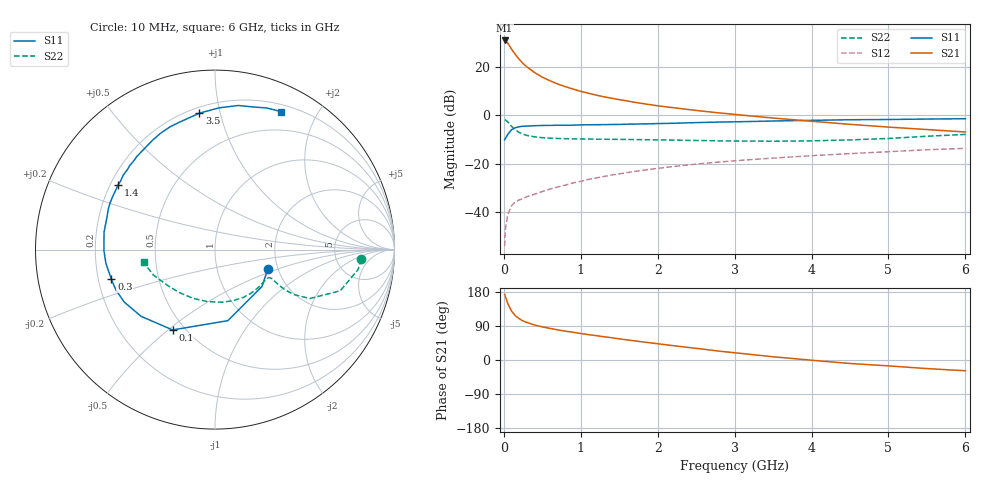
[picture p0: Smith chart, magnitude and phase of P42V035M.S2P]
! SIEMENS Small Signal Semiconductors
! BFP182
! Si NPN RF Bipolar Junction Transistor in SOT143
! VCE = 2 V  IC = 35 mA
! Common Emitter S-Parameters:  March  1996
# GHz  S  MA  R  50
!  f  S11  S21  S12  S22
! GHz  MAG  ANG  MAG  ANG  MAG  ANG  MAG  ANG
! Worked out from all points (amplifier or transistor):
!   36 points, 10 MHz to 6 GHz, reference 50 ohm
!   highest |S21| = 30.9 dB at 10 MHz (marker M1)
!   |S21| within 3 dB of that: start of sweep to 89.2 MHz
!   unconditionally stable (mu >= 1): start of sweep to 20.37 MHz; 224.8 MHz to end of sweep
!   at 250 MHz: K = 1.08, MAG = 26.2 dB, |S12| = -34.3 dB
!   at 1.4 GHz: K = 1.82, MAG = 10.6 dB, |S12| = -24.6 dB
!   at 6 GHz: K = 1.28, MAG = 0.2 dB, |S12| = -13.6 dB
!   S11 on the Smith chart (normalised r, x): 10 MHz: 1.77, -0.42; 100 MHz: 0.43, -0.52; 300 MHz: 0.25, -0.13; 1.4 GHz: 0.23, +0.29; 3.5 GHz: 0.24, +0.86; 6 GHz: 0.28, +1.55
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0.01  0.3135 -19.8  35.15 173.4  0.002 73.6  0.8155 -3.7
0.02  0.3328 -38.0  34.93 167.2  0.0044 75.7  0.8051 -7.9
0.05  0.4022 -79.7  31.15 149.4  0.0089 67.6  0.7348 -18.2
0.1  0.5061 -117.8  23.39 129.1  0.0136 50.9  0.5944 -27.3
0.15  0.5547 -137.9  17.98 116.8  0.0165 46.7  0.5017 -29.8
0.2  0.5843 -150.0  14.3 108.9  0.018 45.1  0.444 -29.8
0.25  0.5964 -158.0  11.77 103.1  0.0192 45.1  0.4086 -29.1
0.3  0.6006 -164.1  10.01 99.1  0.021 46.1  0.3859 -28.3
0.4  0.6126 -172.8  7.652 92.4  0.0236 50.4  0.3602 -27.2
0.5  0.6189 -179.4  6.141 87.5  0.0268 51.8  0.3465 -27.0
0.6  0.6208 175.2  5.179 83.3  0.0302 54.9  0.3384 -27.5
0.7  0.6258 171.0  4.434 79.6  0.0333 56.0  0.334 -28.5
0.8  0.6257 167.1  3.915 76.1  0.0364 57.7  0.3306 -29.8
1.1  0.6397 156.0  2.862 66.9  0.0477 58.6  0.3243 -34.7
1.4  0.6487 146.5  2.263 58.8  0.0587 58.4  0.3205 -40.5
1.8  0.6666 135.4  1.757 47.9  0.0732 56.5  0.3156 -49.4
2.2  0.6864 124.9  1.441 37.8  0.0879 53.5  0.31 -59.2
2.8  0.7284 110.2  1.124 23.3  0.1089 48.2  0.2977 -75.8
3.5  0.7648 96.6  0.881 8.5  0.1315 41.4  0.2927 -97.7
4.5  0.8131 80.9  0.653 -9.2  0.1625 31.9  0.3117 -130.1
5.5  0.8403 69.9  0.51 -22.6  0.1956 22.3  0.3712 -157.6
6  0.852 64.5  0.454 -28.4  0.2082 16.7  0.4045 -169.8
